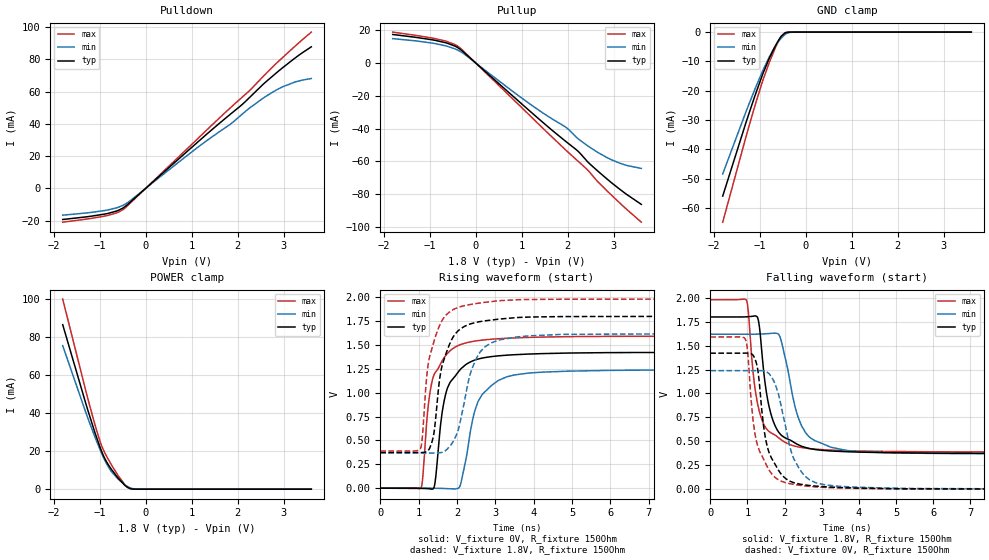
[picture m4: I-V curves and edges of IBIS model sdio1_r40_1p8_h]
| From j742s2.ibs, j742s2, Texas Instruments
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|   r40_1p8_h
[Model]   sdio1_r40_1p8_h
Model_type   I/O
Polarity   Non-Inverting
Enable   Active-High
Vinl = 0
Vinh = 0.8
Vmeas = 0.9
Vref = 1.8
Cref = 2pF
Rref = 100000
|   typ   min   max
C_comp   4.211pF   3.802pF   4.537pF
[Voltage Range]   1.8   1.62   1.98
[Temperature Range]   27   150   -40
[Pullup Reference]   1.8   1.62   1.98
[Pulldown Reference]   0   0   0
[Power Clamp Reference]   1.8   1.62   1.98
[GND Clamp Reference]   0   0   0
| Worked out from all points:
|   slope of the pulldown table from 0 to 0.27 V, typ, clamps not added: 39.2 ohm
|   slope of the pullup table from 0 to 0.27 V, typ, clamps not added: 39.9 ohm
|   GND clamp passes 1 mA (typ) near -0.50 V on its own axis
|   POWER clamp passes 1 mA (typ) near -0.39 V on its own axis
|   falling waveform, V_fixture 1.8V, R_fixture 150Ohm: 20-80 % time 381ps typ, 505ps min, 345ps max; typ from 1.8 V to 0.374 V
|   rising waveform, V_fixture 0V, R_fixture 150Ohm: 20-80 % time 392ps typ, 476ps min, 388ps max; typ from 0 V to 1.42 V
|   rising waveform, V_fixture 1.8V, R_fixture 150Ohm: 20-80 % time 390ps typ, 483ps min, 375ps max; typ from 0.374 V to 1.8 V
|   falling waveform, V_fixture 0V, R_fixture 150Ohm: 20-80 % time 395ps typ, 510ps min, 391ps max; typ from 1.42 V to 0 V
[Pulldown]
|   Voltage   I(typ)   I(min)   I(max)
-1.8V     -19.28mA   -16.58mA   -20.93mA
-892.8mV  -15.94mA   -13.72mA   -17.19mA
-622.8mV  -13.96mA   -11.96mA   -15.1mA
-498.6mV  -12.28mA   -10.57mA   -13.28mA
-298.8mV  -7.64mA    -6.833mA   -8.173mA
1.154V    29.3mA     25.93mA    31.47mA
1.856V    46.38mA    40.15mA    50.39mA
2.12V     52.65mA    46.63mA    57.18mA
2.552V    64.58mA    55.99mA    69.41mA
2.968V    74.7mA     62.95mA    81mA
3.292V    81.89mA    66.42mA    89.43mA
3.6V      87.86mA    68.2mA     97mA
[GND Clamp]
|   Voltage   I(typ)   I(min)   I(max)
-1.8V     -55.9mA    -48.35mA   -64.79mA
-1.287V   -30.48mA   -26.87mA   -35.27mA
-1.109V   -22.12mA   -19.8mA    -25.59mA
-946.8mV  -15.01mA   -13.77mA   -17.35mA
-790.2mV  -8.997mA   -8.533mA   -10.48mA
-622.8mV  -3.762mA   -4.011mA   -4.148mA
-541.8mV  -1.721mA   -2.298mA   -1.693mA
-450mV    -363uA     -857.5uA   -221.7uA
-347.4mV  -20.25uA   -138.5uA   -4.047uA
-234mV    -328.7nA   -10.21uA   -105.1nA
3.6V      0A         0A         0A
[Pullup]
|   Voltage   I(typ)   I(min)   I(max)
-1.8V     17.29mA    14.76mA    18.75mA
-887.4mV  13.77mA    11.79mA    14.82mA
-628.2mV  12.1mA     10.22mA    13.07mA
-363.6mV  8.839mA    7.421mA    9.688mA
1.138V    -28.35mA   -24.18mA   -30.97mA
1.969V    -48.05mA   -39.37mA   -53.35mA
2.201V    -53.23mA   -45.58mA   -59.29mA
2.434V    -60.24mA   -50.5mA    -65.2mA
2.639V    -65.53mA   -54.28mA   -71.94mA
2.866V    -70.99mA   -57.86mA   -78.26mA
3.13V     -76.95mA   -61.09mA   -85.31mA
3.6V      -86.2mA    -64.31mA   -97.05mA
[POWER Clamp]
|   Voltage   I(typ)   I(min)   I(max)
-1.8V     86.44mA    75.43mA    99.9mA
-1.287V   44.12mA    39.56mA    50.59mA
-1.109V   30.39mA    27.98mA    34.62mA
-984.6mV  21.72mA    20.51mA    24.79mA
-898.2mV  16.68mA    15.82mA    19.69mA
-741.6mV  10.42mA    9.224mA    12.8mA
-595.8mV  5.776mA    5.267mA    7.057mA
-450mV    2.018mA    2.285mA    2.308mA
-390.6mV  933uA      1.359mA    950.1uA
-320.4mV  226.3uA    591.6uA    146.8uA
-147.6mV  917.5nA    14.06uA    197.8nA
3.6V      0A         0A         0A
[Ramp]
R_load = 150
|   typ   min   max
dV/dt_r   0.852598/3.91919e-10   0.742887/4.76013e-10   0.954205/3.88609e-10
dV/dt_f   0.855747/3.79521e-10   0.751111/5.00023e-10   0.954658/3.44802e-10
[Falling Waveform]
V_fixture = 1.8V
V_fixture_min = 1.62V
V_fixture_max = 1.98V
R_fixture = 150Ohm
C_fixture = 0F
|   Time   V(typ)   V(min)   V(max)
0s        1.8V       1.62V      1.98V
970ps     1.802V     1.62V      1.978V
1.26ns    1.802V     1.62V      919.6mV
1.495ns   1.052V     1.624V     640.3mV
1.63ns    788.7mV    1.628V     589.9mV
1.87ns    581.3mV    1.599V     527.6mV
2.14ns    514.9mV    1.137V     466.7mV
2.57ns    434.7mV    587.5mV    428.4mV
3.25ns    399mV      437.8mV    408.3mV
10ns      373.6mV    367.7mV    388.8mV
[Rising Waveform]
V_fixture = 0V
V_fixture_min = 0V
V_fixture_max = 0V
R_fixture = 150Ohm
C_fixture = 0F
|   Time   V(typ)   V(min)   V(max)
0s        269.3uV    665.7uV    176.7uV
1.065ns   -1.958mV   469.1uV    3.076mV
1.11ns    -2.732mV   473.5uV    125.1mV
1.25ns    -5.339mV   427.9uV    861.2mV
1.385ns   -4.684mV   -581.5uV   1.169V
1.67ns    922.7mV    -3.461mV   1.37V
2.075ns   1.237V     18.85mV    1.5V
2.545ns   1.351V     902.5mV    1.545V
3.28ns    1.392V     1.163V     1.569V
10ns      1.421V     1.239V     1.591V
[Rising Waveform]
V_fixture = 1.8V
V_fixture_min = 1.62V
V_fixture_max = 1.98V
R_fixture = 150Ohm
C_fixture = 0F
|   Time   V(typ)   V(min)   V(max)
0s        373.6mV    367.7mV    388.8mV
1.045ns   372.7mV    367.4mV    412.9mV
1.095ns   373.3mV    367.4mV    526mV
1.27ns    406.1mV    367.3mV    1.346V
1.4ns     578.6mV    367.2mV    1.536V
1.605ns   1.272V     374.5mV    1.751V
1.975ns   1.625V     548.6mV    1.884V
2.49ns    1.735V     1.346V     1.932V
3.08ns    1.769V     1.549V     1.962V
10ns      1.8V       1.62V      1.98V
[Falling Waveform]
|Gnd
V_fixture = 0V
V_fixture_min = 0V
V_fixture_max = 0V
R_fixture = 150Ohm
C_fixture = 0F
|   Time   V(typ)   V(min)   V(max)
0s        1.421V     1.239V     1.591V
945ps     1.422V     1.239V     1.567V
1.01ns    1.422V     1.239V     1.42V
1.17ns    1.389V     1.239V     666.5mV
1.28ns    1.244V     1.239V     447.9mV
1.525ns   459.3mV    1.224V     241.5mV
1.93ns    147.1mV    825.9mV    80.49mV
2.25ns    67.74mV    316.5mV    49.84mV
2.87ns    31.49mV    63.8mV     23.15mV
10ns      269.3uV    665.9uV    178.1uV
